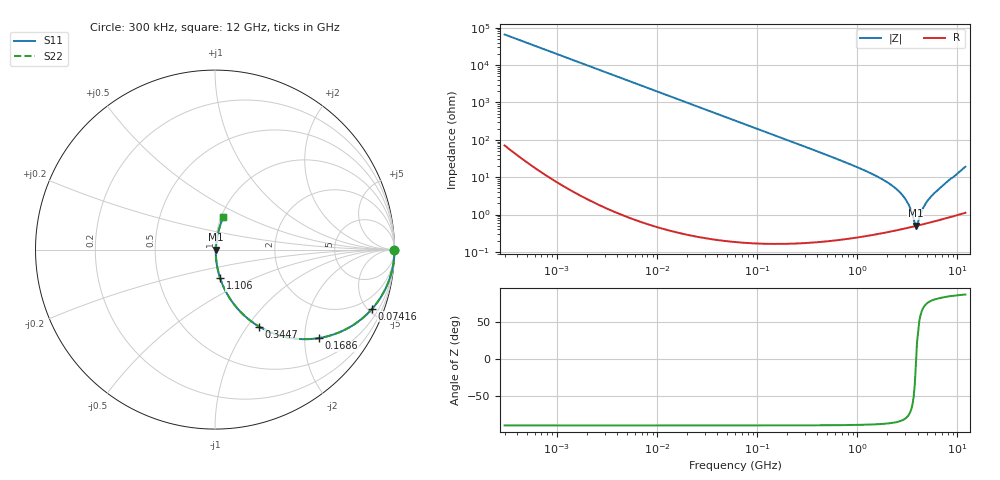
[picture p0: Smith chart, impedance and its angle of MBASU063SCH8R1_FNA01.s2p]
! MBASU063SCH8R1_FNA01  S-PARAMETER MODEL  ( General Type )
! Model Generated by TAIYO YUDEN Corporation (http://www.ty-top.com)
! Version 1.0
! TAIYO YUDEN Control No. 130801
! Copyright(c) 2013 TAIYO YUDEN CO.,LTD. All Rights Reserved.
! Product Description (link to TY-COMPAS)
! https://ds.yuden.co.jp/TYCOMPAS/or/detail?pn=MBASU063SCH8R1DFNA01&u=M
! Products Name : Multilayer Ceramic Capacitors
! Characteristics :
!  Capacitance : 8.1 pF , Rated Voltage : 50V , TCC : CH / C0H
!  Case Size : 0.6 x 0.3 / 0.024 x 0.012 [mm/inch] , Thickness : 0.3 / 0.012 [mm/inch]
!  (Conditions: Temperature = 25 degC , DC Bias Current/Voltage = 0A / 0V)
! External Node Assignments :
!  1  o---| |---o  2
! GND o---------o GND
! Frequency Range : 0.3MHz  -  12000MHz  [ 401 STEP ]
# MHz S RI R 50
! Freq[MHz].  S11 Real  S11 Imag  S21 Real  S21 Imag  S12 Real  S12 Imag  S22 Real  S22 Imag
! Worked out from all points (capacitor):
!   401 points, 300 kHz to 12 GHz, reference 50 ohm
!   read as one part in series: C = 8.06 pF near 316.3 kHz
!   lowest |Z| = 500 mohm at 3.841 GHz (marker M1)
!   series resonance near 3.869 GHz, so ESL is about 210 pH
!   S11 on the Smith chart (normalised r, x): 300 kHz: open; 74.16 MHz: 1.00, -5.33; 168.6 MHz: 1.00, -2.34; 344.7 MHz: 1.00, -1.14; 1.106 GHz: 1.01, -0.33; 12 GHz: 1.02, +0.38
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0.3  1 -0.00152  3.93e-06 0.00152  3.93e-06 0.00152  1 -0.00152
1.769972  0.9999 -0.00896  8.27e-05 0.00896  8.27e-05 0.00896  0.9999 -0.00896
10.44266  0.9972 -0.0527  0.0028 0.0527  0.0028 0.0527  0.9972 -0.0527
27.10171  0.9815 -0.1346  0.0185 0.1346  0.0185 0.1346  0.9815 -0.1346
60  0.9154 -0.278  0.0846 0.278  0.0846 0.278  0.9154 -0.278
74.16388  0.8762 -0.329  0.1238 0.329  0.1238 0.329  0.8762 -0.329
168.5979  0.5775 -0.4933  0.4225 0.4933  0.4225 0.4933  0.5775 -0.4933
344.7396  0.2449 -0.4285  0.7551 0.4285  0.7551 0.4285  0.2449 -0.4285
353.9943  0.2352 -0.4225  0.7648 0.4225  0.7648 0.4225  0.2352 -0.4225
585.5907  0.0995 -0.2963  0.9005 0.2963  0.9005 0.2963  0.0995 -0.2963
1105.905  0.0285 -0.159  0.9715 0.159  0.9715 0.159  0.0285 -0.159
2088.533  0.00787 -0.0663  0.9921 0.0663  0.9921 0.0663  0.00787 -0.0663
2581.562  0.00565 -0.0421  0.9944 0.0421  0.9944 0.0421  0.00565 -0.0421
3026.31  0.00488 -0.0252  0.9951 0.0252  0.9951 0.0252  0.00488 -0.0252
3276.641  0.00474 -0.017  0.9953 0.017  0.9953 0.017  0.00474 -0.017
3642.919  0.00479 -0.00616  0.9952 0.00616  0.9952 0.00616  0.00479 -0.00616
3841.137  0.00491 -0.000752  0.9951 0.000752  0.9951 0.000752  0.00491 -0.000752
4050.141  0.0051 0.00373  0.9949 -0.00373  0.9949 -0.00373  0.0051 0.00373
4623.766  0.00577 0.0152  0.9942 -0.0152  0.9942 -0.0152  0.00577 0.0152
5278.635  0.00676 0.0266  0.9932 -0.0266  0.9932 -0.0266  0.00676 0.0266
8064.993  0.0142 0.0774  0.9858 -0.0774  0.9858 -0.0774  0.0142 0.0774
12000  0.0446 0.1792  0.9554 -0.1792  0.9554 -0.1792  0.0446 0.1792
